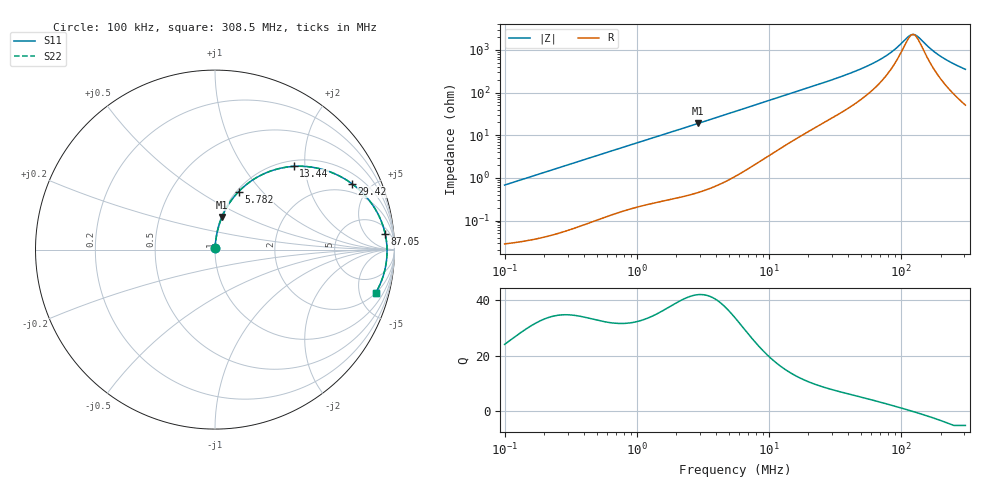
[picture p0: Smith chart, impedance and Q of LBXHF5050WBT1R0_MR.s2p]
! LBXHF5050WBT1R0_MR  S-PARAMETER MODEL  ( General Type )
! Model Generated by TAIYO YUDEN Corporation (http://www.ty-top.com)
! Version 1.0
! TAIYO YUDEN Control No. 210719NI43SB-FBB
! Copyright(c) 2021 TAIYO YUDEN CO.,LTD. All Rights Reserved.
! Product Description (link to TY-COMPAS)
! https://ds.yuden.co.jp/TYCOMPAS/or/detail?pn=LBXHF5050WBT1R0NMR&u=M
! Products Name : Inductors
! Characteristics :
!  Inductance : 1.0 uH , SRF(min) : 85 MHz , DC Resistance(max) : 0.024 Ohm
!  Rated Current : Saturation :5000 mA , Temp Rise : 2600 mA
!  Case Size : 5.0 x 5.0 / 0.197 x 0.197 [mm/inch] , Thickness : 2.2 / 0.087 [mm/inch]
!  (Conditions: Temperature = 25 degC , DC Bias Current/Voltage = 0A / 0V)
! External Node Assignments :
!  1  o---GGG---o  2
! GND o---------o GND
! Frequency Range : 0.1MHz  -  308.54851MHz  [ 402 STEP ]
# MHz S RI R 50
! Freq[MHz].  S11 Real  S11 Imag  S21 Real  S21 Imag  S12 Real  S12 Imag  S22 Real  S22 Imag
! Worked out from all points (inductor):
!   401 points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, 100 kHz to 308.5 MHz, reference 50 ohm
!   read as one part in series: L = 1.08 uH near 104.1 kHz
!   highest Q = 41.8 at 2.921 MHz (marker M1), where L = 1.03 uH
!   self-resonance near 123.6 MHz
!   S11 on the Smith chart (normalised r, x): 100 kHz: 1.00, +0.01; 5.782 MHz: 1.02, +0.75; 13.44 MHz: 1.12, +1.75; 29.42 MHz: 1.49, +3.86; 87.05 MHz: 9, +17; 308.5 MHz: 2.02, -6.96
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0.1  0.000329 0.00678  0.9997 -0.00678  0.9997 -0.00678  0.000329 0.00678
0.384115  0.00142 0.0257  0.9986 -0.0257  0.9986 -0.0257  0.00142 0.0257
1.475446  0.0118 0.0949  0.9882 -0.0949  0.9882 -0.0949  0.0118 0.0949
2.920894  0.0387 0.1812  0.9613 -0.1812  0.9613 -0.1812  0.0387 0.1812
5.667415  0.1267 0.3178  0.8733 -0.3178  0.8733 -0.3178  0.1267 0.3178
5.782403  0.1311 0.3225  0.8689 -0.3225  0.8689 -0.3225  0.1311 0.3225
8.641209  0.2497 0.4114  0.7503 -0.4114  0.7503 -0.4114  0.2497 0.4114
13.44272  0.438 0.4637  0.562 -0.4637  0.562 -0.4637  0.438 0.4637
21.33651  0.6462 0.4312  0.3538 -0.4312  0.3538 -0.4312  0.6462 0.4312
29.42364  0.764 0.3664  0.236 -0.3664  0.236 -0.3664  0.764 0.3664
53.75212  0.9017 0.2106  0.0983 -0.2106  0.0983 -0.2106  0.9017 0.2106
67.04278  0.9287 0.1527  0.0713 -0.1527  0.0713 -0.1527  0.9287 0.1527
81.95682  0.945 0.1015  0.055 -0.1015  0.055 -0.1015  0.945 0.1015
87.04724  0.9485 0.0864  0.0515 -0.0864  0.0515 -0.0864  0.9485 0.0864
115.3138  0.9579 0.017  0.0421 -0.017  0.0421 -0.017  0.9579 0.017
122.4761  0.9585 0.00224  0.0415 -0.00224  0.0415 -0.00224  0.9585 0.00224
127.4964  0.9586 -0.00763  0.0414 0.00763  0.0414 0.00763  0.9586 -0.00763
135.4153  0.9584 -0.0225  0.0416 0.0225  0.0416 0.0225  0.9584 -0.0225
168.8979  0.9533 -0.0778  0.0467 0.0778  0.0467 0.0778  0.9533 -0.0778
198.3402  0.9449 -0.1193  0.0551 0.1193  0.0551 0.1193  0.9449 -0.1193
247.3814  0.9257 -0.1791  0.0743 0.1791  0.0743 0.1791  0.9257 -0.1791
308.5485  0.8952 -0.2418  0.1048 0.2418  0.1048 0.2418  0.8952 -0.2418
